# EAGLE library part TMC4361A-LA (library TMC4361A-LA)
S-ramp motion controller for stepper motors with high velocities. With SPI and Step/Dir; QFN40(5x5)
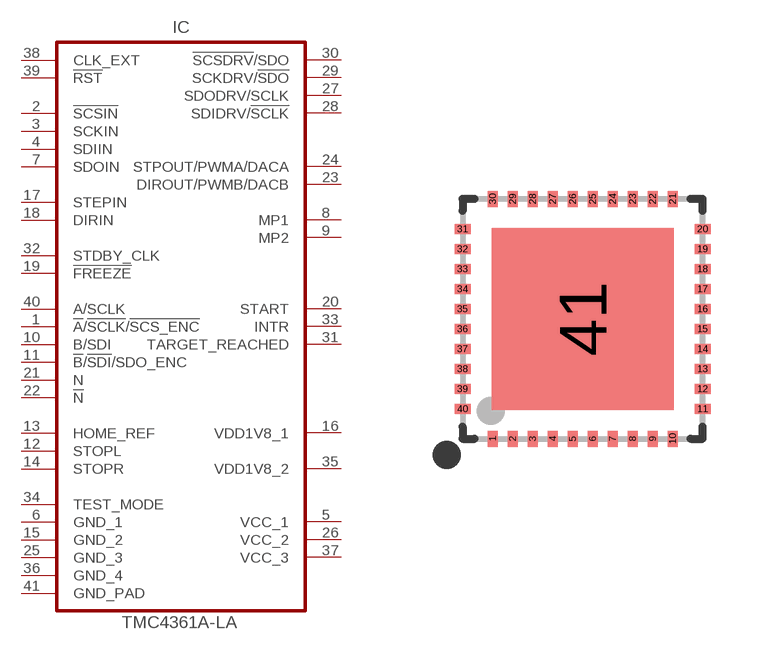
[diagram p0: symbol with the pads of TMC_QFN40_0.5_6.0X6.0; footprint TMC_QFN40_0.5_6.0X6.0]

Designator prefix IC

## TMC4361A-LA (DESCRIPTION: S-ramp motion controller for stepper motors with high velocities_ With SPI and Step/Dir; QFN40(5x5); GEOMETRY_HEIGHT: 0_9mm; MANUFACTURER: TRINAMIC; ORDERCODE-MANU1: TMC4361A-LA; VALUE: TMC4361A-LA)  [TMC_QFN40_0.5_6.0X6.0]
1  !A!/!SCLK!/!SCS_ENC
2  !SCSIN!  in
3  SCKIN  in
4  SDIIN  in
5  VCC_1  pwr
6  GND_1  pwr
7  SDOIN  out
8  MP1
9  MP2
10  B/SDI  in
11  !B!/!SDI!/SDO_ENC
12  STOPL  in
13  HOME_REF  in
14  STOPR  in
15  GND_2  pwr
16  VDD1V8_1  pwr
17  STEPIN  in
18  DIRIN  in
19  !FREEZE!  in
20  START
21  N  in
22  !N!  in
23  DIROUT/PWMB/DACB  out
24  STPOUT/PWMA/DACA  out
25  GND_3  pwr
26  VCC_2  pwr
27  SDODRV/SCLK
28  SDIDRV/!SCLK!  in
29  SCKDRV/!SDO!  out
30  !SCSDRV!/SDO  out
31  TARGET_REACHED  out
32  STDBY_CLK  out
33  INTR  out
34  TEST_MODE  in
35  VDD1V8_2  pwr
36  GND_4  pwr
37  VCC_3  pwr
38  CLK_EXT  in
39  !RST!  in
40  A/SCLK
41  GND_PAD  pwr

## Footprint TMC_QFN40_0.5_6.0X6.0 (pad centres in mm)
smd 0.25 x 0.4: 1 -2.25,-3; 2 -1.75,-3; 3 -1.25,-3; 4 -0.75,-3; 5 -0.25,-3; 6 0.25,-3; 7 0.75,-3; 8 1.25,-3; 9 1.75,-3; 10 2.25,-3; 21 2.25,3; 22 1.75,3; 23 1.25,3; 24 0.75,3; 25 0.25,3; 26 -0.25,3; 27 -0.75,3; 28 -1.25,3; 29 -1.75,3; 30 -2.25,3
smd 0.4 x 0.25: 11 3,-2.25; 12 3,-1.75; 13 3,-1.25; 14 3,-0.75; 15 3,-0.25; 16 3,0.25; 17 3,0.75; 18 3,1.25; 19 3,1.75; 20 3,2.25; 31 -3,2.25; 32 -3,1.75; 33 -3,1.25; 34 -3,0.75; 35 -3,0.25; 36 -3,-0.25; 37 -3,-0.75; 38 -3,-1.25; 39 -3,-1.75; 40 -3,-2.25
smd 4.55 x 4.55: 41 0,0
